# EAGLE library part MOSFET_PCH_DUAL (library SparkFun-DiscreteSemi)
Dual P-Channel -20VDS MOSFET Link to datasheet SparkFun Products: SparkFun FreeSoC2 Development Board
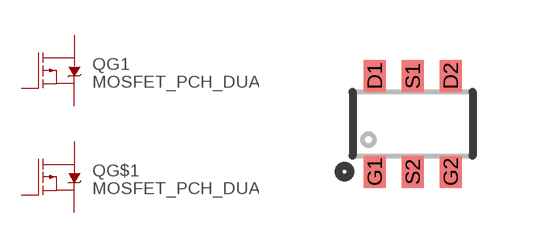
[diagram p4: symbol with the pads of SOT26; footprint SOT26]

Designator prefix Q; gates G1=LABELED-PMOS G$1=LABELED-PMOS

## MOSFET_PCH_DUAL-DMP2240UDM (PROD_ID: TRANS-12444; VALUE: 2A/20V/150mΩ)  [SOT26]
D1  G1:D
D2  G$1:D
G1  G1:G
G2  G$1:G
S1  G1:S
S2  G$1:S

## Footprint SOT26 (pad centres in mm)
Footprint for SOT-26 part DMP2240UDM
smd 0.55 x 0.8: D1 -0.95,1.2; D2 0.95,1.2; G1 -0.95,-1.2; G2 0.95,-1.2; S1 0,1.2; S2 0,-1.2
